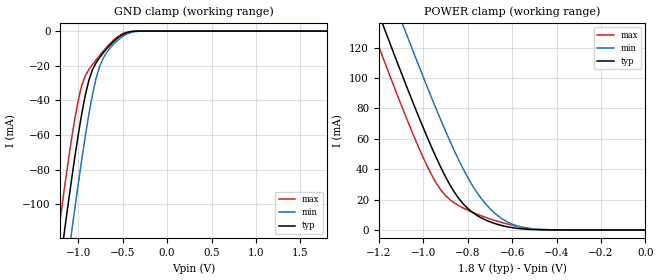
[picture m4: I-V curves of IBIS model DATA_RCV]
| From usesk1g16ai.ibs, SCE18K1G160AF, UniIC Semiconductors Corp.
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|   Model DATA_RCV
[Model]  DATA_RCV
Model_type Input
Polarity   Non-Inverting
Vinl = 360.000mV
Vinh = 1440.000mV
C_comp   2.0990pF   2.0750pF   2.3110pF
[Temperature Range]   25.0000   85.0000   -40.0000
[Voltage Range]   1.8000V   1.7000V   1.9000V
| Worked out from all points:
|   GND clamp passes 1 mA (typ) near -0.46 V on its own axis
|   POWER clamp passes 1 mA (typ) near -0.57 V on its own axis
[GND_clamp]
|Voltage   I(typ)   I(min)   I(max)
-1.8V     -382.1mA   -414.5mA   -357.5mA
-1.24V    -149mA     -181.4mA   -123.6mA
-1.2V     -133.2mA   -165.3mA   -107.9mA
-1.16V    -117.7mA   -149.4mA   -92.62mA
-1.08V    -87.61mA   -118.3mA   -63.92mA
-960mV    -47.64mA   -74.16mA   -31.42mA
-880mV    -28.39mA   -48.02mA   -22.22mA
-800mV    -18.4mA    -27.56mA   -16.75mA
-680mV    -10.16mA   -12.34mA   -9.318mA
-520mV    -2.567mA   -3.816mA   -2.005mA
-280mV    -6.329uA   -40.92uA   -4.704uA
1.8V      3.312nA    86.13nA    479.4pA
[POWER_clamp]
|Voltage   I(typ)   I(min)   I(max)
-1.8V     384.7mA    419.1mA    364.2mA
-1.24V    157.9mA    192.8mA    136.4mA
-1.22V    150.1mA    184.9mA    128.5mA
-1.18V    134.5mA    169.2mA    113mA
-1.16V    126.8mA    161.4mA    105.2mA
-1.08V    96.37mA    130.6mA    75.23mA
-980mV    60.39mA    93.37mA    41.35mA
-900mV    35.09mA    65.23mA    22.71mA
-800mV    14.21mA    34.63mA    13.04mA
-680mV    4.343mA    11.31mA    6.353mA
-520mV    368.6uA    1.001mA    926.5uA
0V        3.312nA    53.68nA    602.9pA
